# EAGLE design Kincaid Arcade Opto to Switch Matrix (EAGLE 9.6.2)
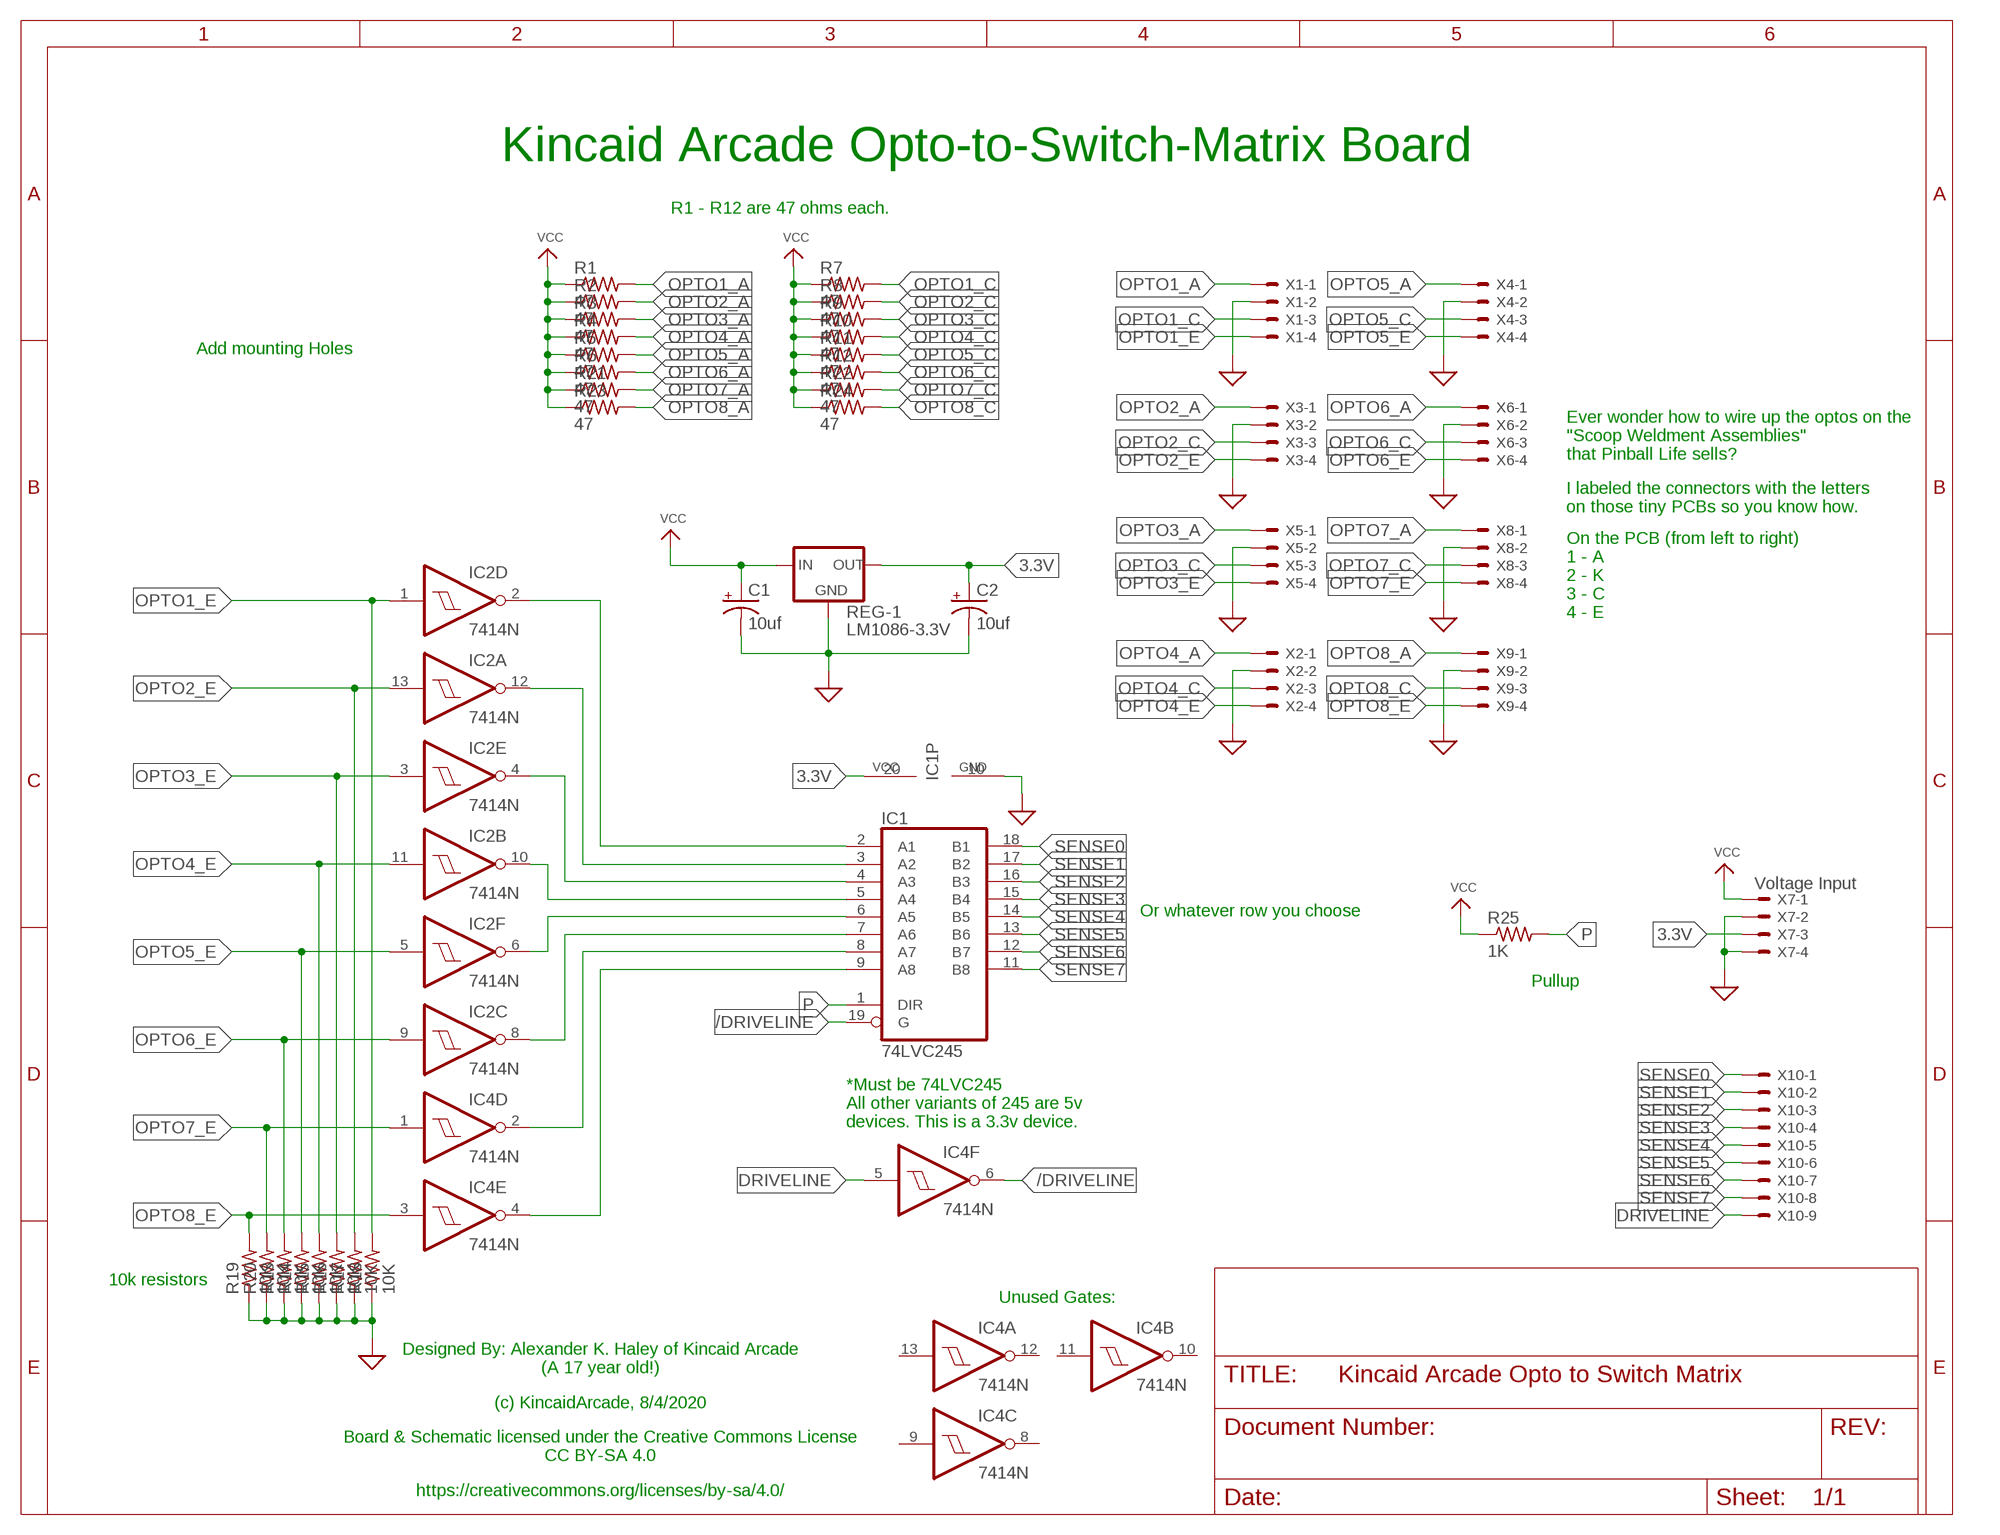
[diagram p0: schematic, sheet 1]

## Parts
C1  10uf  CPOL-USB45181A  [B45181A]
C2  10uf  CPOL-USB45181A  [B45181A]
IC1  74LVC245  74LS245N  [DIL20]
IC2  7414N  [DIL14]
IC4  7414N  [DIL14]
R1  47  R-US_0207/7  [0207/7]
R2  47  R-US_0207/7  [0207/7]
R3  47  R-US_0207/7  [0207/7]
R4  47  R-US_0207/7  [0207/7]
R5  47  R-US_0207/7  [0207/7]
R6  47  R-US_0207/7  [0207/7]
R7  47  R-US_0207/7  [0207/7]
R8  47  R-US_0207/7  [0207/7]
R9  47  R-US_0207/7  [0207/7]
R10  47  R-US_0207/7  [0207/7]
R11  47  R-US_0207/7  [0207/7]
R12  47  R-US_0207/7  [0207/7]
R13  10K  R-US_0207/7  [0207/7]
R14  10K  R-US_0207/7  [0207/7]
R15  10K  R-US_0207/7  [0207/7]
R16  10K  R-US_0207/7  [0207/7]
R17  10K  R-US_0207/7  [0207/7]
R18  10K  R-US_0207/7  [0207/7]
R19  10K  R-US_0207/7  [0207/7]
R20  10K  R-US_0207/7  [0207/7]
R21  47  R-US_0207/7  [0207/7]
R22  47  R-US_0207/7  [0207/7]
R23  47  R-US_0207/7  [0207/7]
R24  47  R-US_0207/7  [0207/7]
R25  1K  R-US_0207/7  [0207/7]
REG-1  LM1086-3.3V  LM1086  [78XXL]
X1  KK-156-4  [KK-156-4]
X2  KK-156-4  [KK-156-4]
X3  KK-156-4  [KK-156-4]
X4  KK-156-4  [KK-156-4]
X5  KK-156-4  [KK-156-4]
X6  KK-156-4  [KK-156-4]
X7  Voltage Input  KK-156-4  [KK-156-4]
X8  KK-156-4  [KK-156-4]
X9  KK-156-4  [KK-156-4]
X10  KK-156-9  [KK-156-9]

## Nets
3.3V: C2.+ IC1.20(VCC) REG-1.OUT X7.3
/DRIVELINE: IC1.19(G) IC4.6(F:O)
DRIVELINE: IC4.5(F:I) X10.9
GND: C1.- C2.- IC1.10(GND) R13.1 R14.1 R15.1 R16.1 R17.1 R18.1 R19.1 R20.1 REG-1.GND X1.2 X2.2 X3.2 X4.2 X5.2 X6.2 X7.2 X7.4 X8.2 X9.2 ; supply symbol labelled SUP
N$1: IC1.9(A8) IC4.4(E:O)
N$2: IC1.8(A7) IC4.2(D:O)
N$3: IC1.7(A6) IC2.8(C:O)
N$4: IC1.6(A5) IC2.6(F:O)
N$5: IC1.5(A4) IC2.10(B:O)
N$6: IC1.4(A3) IC2.4(E:O)
N$7: IC1.3(A2) IC2.12(A:O)
N$8: IC1.2(A1) IC2.2(D:O)
OPTO1_A: R1.2 X1.1
OPTO1_C: R7.2 X1.3
OPTO1_E: IC2.1(D:I) R18.2 X1.4
OPTO2_A: R2.2 X3.1
OPTO2_C: R8.2 X3.3
OPTO2_E: IC2.13(A:I) R17.2 X3.4
OPTO3_A: R3.2 X5.1
OPTO3_C: R9.2 X5.3
OPTO3_E: IC2.3(E:I) R16.2 X5.4
OPTO4_A: R4.2 X2.1
OPTO4_C: R10.2 X2.3
OPTO4_E: IC2.11(B:I) R15.2 X2.4
OPTO5_A: R5.2 X4.1
OPTO5_C: R11.2 X4.3
OPTO5_E: IC2.5(F:I) R14.2 X4.4
OPTO6_A: R6.2 X6.1
OPTO6_C: R12.2 X6.3
OPTO6_E: IC2.9(C:I) R13.2 X6.4
OPTO7_A: R21.2 X8.1
OPTO7_C: R22.2 X8.3
OPTO7_E: IC4.1(D:I) R20.2 X8.4
OPTO8_A: R23.2 X9.1
OPTO8_C: R24.2 X9.3
OPTO8_E: IC4.3(E:I) R19.2 X9.4
P: IC1.1(DIR) R25.2
SENSE0: IC1.18(B1) X10.1
SENSE1: IC1.17(B2) X10.2
SENSE2: IC1.16(B3) X10.3
SENSE3: IC1.15(B4) X10.4
SENSE4: IC1.14(B5) X10.5
SENSE5: IC1.13(B6) X10.6
SENSE6: IC1.12(B7) X10.7
SENSE7: IC1.11(B8) X10.8
VCC: C1.+ R1.1 R2.1 R3.1 R4.1 R5.1 R6.1 R7.1 R8.1 R9.1 R10.1 R11.1 R12.1 R21.1 R22.1 R23.1 R24.1 R25.1 REG-1.IN X7.1
Unconnected: IC4.8(C:O) IC4.9(C:I) IC4.10(B:O) IC4.11(B:I) IC4.12(A:O) IC4.13(A:I)

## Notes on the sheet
- Kincaid Arcade Opto-to-Switch-Matrix Board
- R1 - R12 are 47 ohms each.
- Add mounting Holes
- Ever wonder how to wire up the optos on the
  "Scoop Weldment Assemblies"
  that Pinball Life sells?
- I labeled the connectors with the letters
  on those tiny PCBs so you know how.
- On the PCB (from left to right)
  1 - A
  2 - K
  3 - C
  4 - E
- Or whatever row you choose
- Pullup
- *Must be 74LVC245
  All other variants of 245 are 5v
  devices. This is a 3.3v device.
- 10k resistors
- Unused Gates:
- Designed By: Alexander K. Haley of Kincaid Arcade
  (A 17 year old!)
- (c) KincaidArcade, 8/4/2020
- Board & Schematic licensed under the Creative Commons License
  CC BY-SA 4.0
- https://creativecommons.org/licenses/by-sa/4.0/

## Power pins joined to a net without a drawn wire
GND: IC2.7(P:GND) IC4.7(P:GND)
VCC: IC2.14(P:VCC) IC4.14(P:VCC)

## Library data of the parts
C1 C2 = rcl:CPOL-US: POLARIZED CAPACITOR, American symbol; SPICEPREFIX: C
IC1 = 74xx-us:74*245: Octal BUS TRANSCEIVER, 3-state
IC2 IC4 = 74xx-us:74*14: Hex schmitt trigger INVERTER
R1-R24 = resistor:R-US_: RESISTOR, American symbol
R25 = rcl:R-US_: RESISTOR, American symbol; SPICEPREFIX: R
REG-1 = OLD AND OBSOLETE ARCADE PARTS:LM1086
X1-X9 = con-molex:KK-156-4: KK 156 HEADER Source: http://www.molex.com/pdm_docs/sd/026604100_sd.pdf; MF: MOLEX; OC_FARNELL: unknown; OC_NEWARK: unknown
X10 = con-molex:KK-156-9: KK 156 HEADER Source: http://www.molex.com/pdm_docs/sd/026604100_sd.pdf; MF: MOLEX; OC_FARNELL: unknown; OC_NEWARK: unknown

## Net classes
0 default: width 0.406 mm, clearance 0.406 mm

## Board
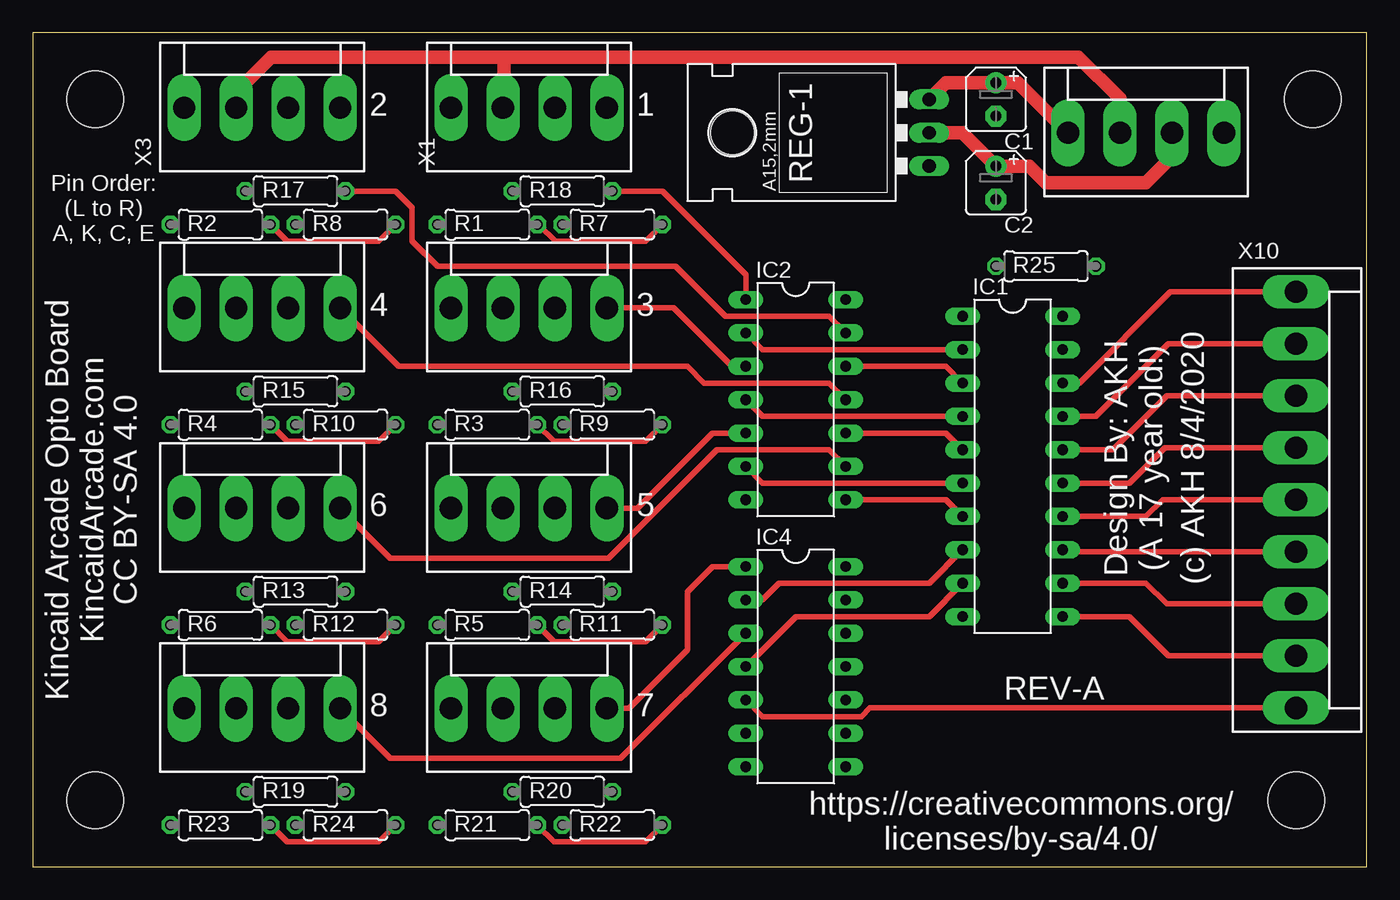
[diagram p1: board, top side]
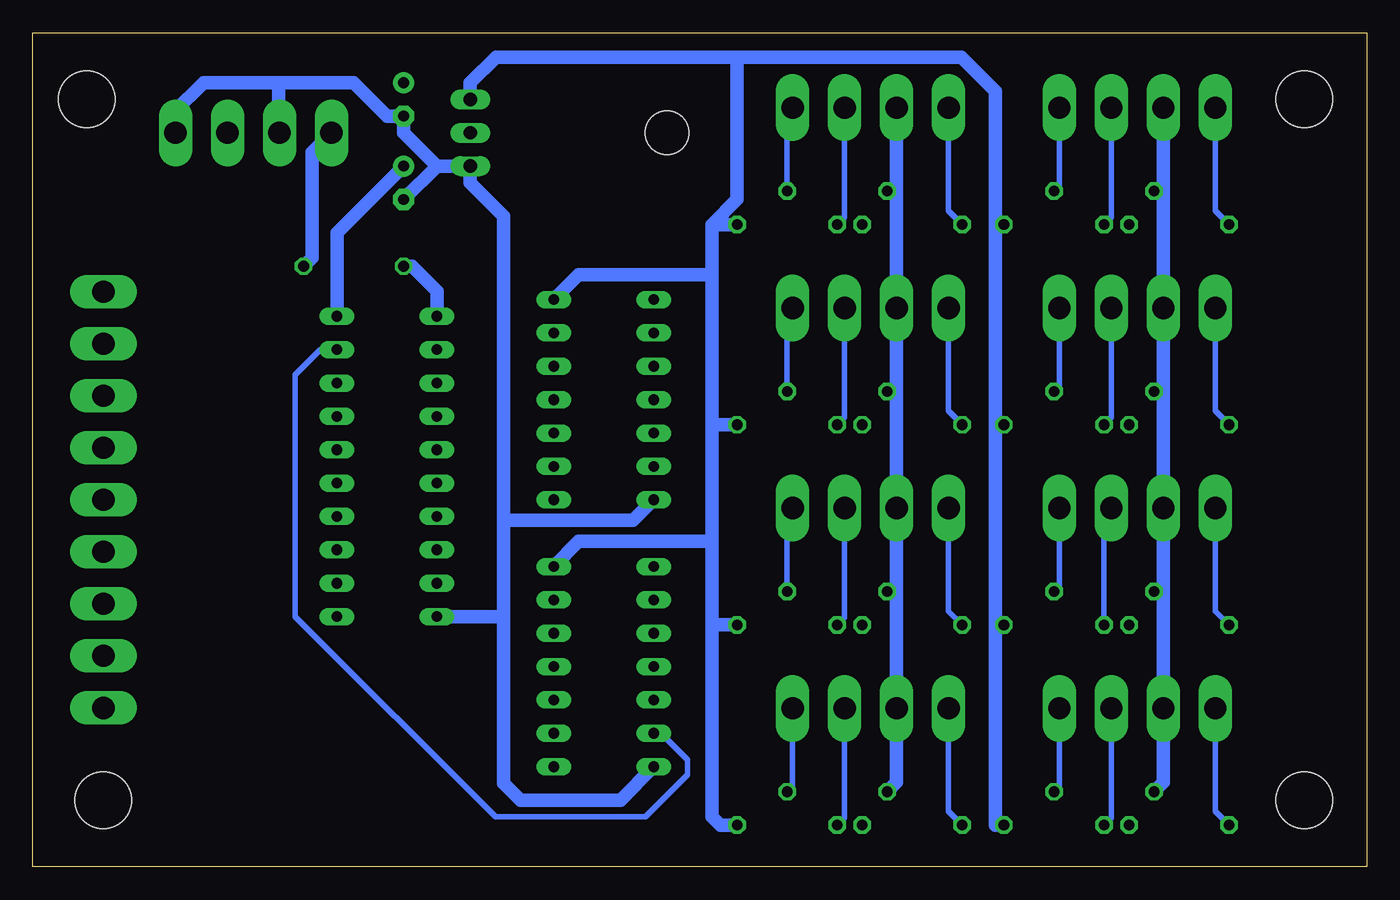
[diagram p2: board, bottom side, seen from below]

Size 101.58 x 63.49 mm. Coordinates in mm from the lower left corner, seen from the top.
Outline: 0,0 101.58,0 101.58,63.49 0,63.49 0,0
Copper layers (1*16): Top 0.035mm / dielectric 1.5mm / Bottom 0.035mm
Design rules "default": minimum track width 6mil, minimum drill 0.35mm, track to track 6mil, track to pad 6mil, pad to pad 6mil, via to via 6mil, smd to smd 6mil, copper to edge 40mil, drill to drill 6mil, minimum pad ring 10mil, minimum via ring 8mil, stop-mask expansion 4mil, vias tented up to drill 0mil, thermal gap 10mil
Holes 4.32 mm at 4.76,58.42 4.76,5.08 97.47,58.42 96.2,5.08

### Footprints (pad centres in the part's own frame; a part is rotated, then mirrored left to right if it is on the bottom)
B45181A = drill 0.813 pad 1.6: + -1.27,0 | drill 0.813 pad 1.6 octagon: - 1.27,0
DIL20 = drill 0.813 long: 1 -11.43,-3.81; 2 -8.89,-3.81; 3 -6.35,-3.81; 4 -3.81,-3.81; 5 -1.27,-3.81; 6 1.27,-3.81; 7 3.81,-3.81; 8 6.35,-3.81; 9 8.89,-3.81; 10 11.43,-3.81; 11 11.43,3.81; 12 8.89,3.81; 13 6.35,3.81; 14 3.81,3.81; 15 1.27,3.81; 16 -1.27,3.81; 17 -3.81,3.81; 18 -6.35,3.81; 19 -8.89,3.81; 20 -11.43,3.81
DIL14 = drill 0.813 long: 1 -7.62,-3.81; 2 -5.08,-3.81; 3 -2.54,-3.81; 4 0,-3.81; 5 2.54,-3.81; 6 5.08,-3.81; 7 7.62,-3.81; 8 7.62,3.81; 9 5.08,3.81; 10 2.54,3.81; 11 0,3.81; 12 -2.54,3.81; 13 -5.08,3.81; 14 -7.62,3.81
0207/7 = drill 0.813 octagon: 1 -3.81,0; 2 3.81,0
78XXL = drill 1.016 long: GND -2.54,-3.81; IN 2.54,-3.81; OUT 0,-3.81 | hole 3.302: 0,11.176
KK-156-4 = drill 1.7 pad 2.184 long: 1 -5.94,0; 2 -1.98,0; 3 1.98,0; 4 5.94,0
KK-156-9 = drill 1.7 pad 2.184 long: 1 -15.84,0; 2 -11.88,0; 3 -7.92,0; 4 -3.96,0; 5 0,0; 6 3.96,0; 7 7.92,0; 8 11.88,0; 9 15.84,0

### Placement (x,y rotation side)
C1  73.34,58.42 270 top
C2  73.34,52.07 270 top
IC1  74.61,30.48 270 top
IC2  58.1,35.56 270 top
IC4  58.1,15.24 270 top
R1  34.61,48.9 180 top
R2  14.29,48.9 180 top
R3  34.61,33.66 180 top
R4  14.29,33.66 180 top
R5  34.61,18.41 180 top
R6  14.29,18.41 180 top
R7  44.13,48.9 180 top
R8  23.81,48.9 180 top
R9  44.13,33.66 180 top
R10  23.81,33.66 180 top
R11  44.13,18.41 180 top
R12  23.81,18.41 180 top
R13  20,20.95 0 top
R14  40.32,20.95 0 top
R15  20,36.2 0 top
R16  40.32,36.2 0 top
R17  20,51.44 0 top
R18  40.32,51.44 0 top
R19  20,5.71 0 top
R20  40.32,5.71 0 top
R21  34.61,3.17 180 top
R22  44.13,3.17 180 top
R23  14.29,3.17 180 top
R24  23.81,3.17 180 top
R25  77.15,45.72 180 top
REG-1  64.45,55.88 90 top
X1  37.78,57.78 0 top
X2  17.46,42.55 0 top
X3  17.46,57.78 0 top
X4  37.78,27.3 0 top
X5  37.78,42.55 0 top
X6  17.46,27.3 0 top
X7  84.77,55.88 0 top
X8  37.78,12.06 0 top
X9  17.46,12.06 0 top
X10  96.2,27.94 270 top

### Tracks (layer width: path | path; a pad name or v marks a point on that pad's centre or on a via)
3.3V
  Top 1.016: REG-1.OUT 70.8,55.88 C2.+ 75.88,53.34 77.15,52.07 84.77,52.07 86.75,54.05 X7.3
  Bottom 1.016: C2.+ 78.42,48.26 IC1.20
/DRIVELINE
  Bottom 0.406: IC4.6 53.74,10.16 51.73,8.15 51.73,7.01 54.93,3.81 66.36,3.81 81.6,19.05 81.6,37.47 79.69,39.37 IC1.19
DRIVELINE
  Top 0.406: X10.9 63.77,12.1 63.1,11.43 55.56,11.43 IC4.5
GND
  Top 1.016: X7.2 82.79,58.49 79.64,61.65 35.88,61.65 | 35.88,61.65 18.15,61.65 15.48,58.98 X3.2 | 35.88,61.65 35.88,57.86 X1.2
  Bottom 1.016: 70.8,53.34 REG-1.GND 68.26,52.07 65.72,49.53 65.72,26.36 | 70.8,53.34 C2.- | 70.8,53.34 73.34,55.88 C1.- 74.61,57.15 77.15,59.69 82.87,59.69 | X7.4 90.85,56.01 90.85,57.43 88.58,59.69 82.87,59.69 | 82.87,59.69 82.87,55.95 X7.2 | 65.72,26.36 65.72,19.05 | 65.72,19.05 65.72,6.35 64.45,5.08 56.83,5.08 IC4.7 | 65.72,26.36 55.87,26.36 IC2.7 | IC1.10 65.72,19.05 | X3.2 15.48,51.44 | 15.48,51.44 X2.2 15.48,36.2 | R17.1 15.48,51.44 | X1.2 35.8,51.44 | 35.8,51.44 X5.2 35.8,36.2 | R18.1 35.8,51.44 | 35.8,36.2 X4.2 35.8,20.95 | R16.1 35.8,36.2 | 15.48,36.2 X6.2 15.48,20.95 | R15.1 15.48,36.2 | 15.48,20.95 X9.2 15.48,6.42 R19.1 | R13.1 15.48,20.95 | 35.8,20.95 X8.2 35.8,6.42 R20.1 | R14.1 35.8,20.95
N$1
  Top 0.406: IC4.4 58.1,19.05 68.26,19.05 IC1.9
N$2
  Top 0.406: IC4.2 55.56,20.32 56.83,21.59 68.26,21.59 IC1.8
N$3
  Top 0.406: IC2.8 69.53,27.94 IC1.7
N$4
  Top 0.406: IC2.6 55.56,29.21 IC1.6
N$5
  Top 0.406: IC2.10 69.53,33.02 IC1.5
N$6
  Top 0.406: IC2.4 55.56,34.29 IC1.4
N$7
  Top 0.406: IC2.12 69.53,38.1 IC1.3
N$8
  Top 0.406: IC2.2 55.56,39.37 IC1.2
OPTO1_A
  Bottom 0.406: X1.1 31.84,49.94 R1.2
OPTO1_C
  Bottom 0.406: X1.3 39.76,49.45 R7.2
OPTO1_E
  Top 0.406: IC2.1 54.29,45.09 47.94,51.44 R18.2
  Bottom 0.406: X1.4 44.13,57.38 R18.2
OPTO2_A
  Bottom 0.406: X3.1 11.52,49.94 R2.2
OPTO2_C
  Bottom 0.406: X3.3 19.44,49.45 R8.2
OPTO2_E
  Top 0.406: IC2.13 60.64,41.91 52.74,41.91 48.95,45.7 30.81,45.7 28.89,47.62 28.89,50.16 27.62,51.44 R17.2
  Bottom 0.406: X3.4 23.4,51.84 R17.2
OPTO3_A
  Bottom 0.406: X5.1 31.84,34.7 R3.2
OPTO3_C
  Bottom 0.406: X5.3 39.76,34.22 R9.2
OPTO3_E
  Top 0.406: X5.4 48.8,42.55 53.25,38.1 IC2.3
  Bottom 0.406: X5.4 44.13,42.13 R16.2
OPTO4_A
  Bottom 0.406: X2.1 11.52,34.7 R4.2
OPTO4_C
  Bottom 0.406: X2.3 19.44,34.22 R10.2
OPTO4_E
  Top 0.406: X2.4 27.85,38.1 49.85,38.1 51.12,36.83 60.64,36.83 IC2.11
  Bottom 0.406: X2.4 23.4,36.6 R15.2
OPTO5_A
  Bottom 0.406: X4.1 31.84,19.46 R5.2
OPTO5_C
  Bottom 0.406: X4.3 39.76,18.98 R11.2
OPTO5_E
  Top 0.406: X4.4 46.04,27.3 51.75,33.02 IC2.5
  Bottom 0.406: X4.4 44.13,26.89 R14.2
OPTO6_A
  Bottom 0.406: X6.1 11.52,19.46 R6.2
OPTO6_C
  Bottom 0.406: X6.3 20,26.75 R12.2
OPTO6_E
  Top 0.406: X6.4 27.21,23.5 43.85,23.5 52.11,31.75 60.64,31.75 IC2.9
  Bottom 0.406: X6.4 23.4,21.36 R13.2
OPTO7_A
  Bottom 0.406: X8.1 31.84,4.22 R21.2
OPTO7_C
  Bottom 0.406: X8.3 39.76,3.73 R22.2
OPTO7_E
  Top 0.406: IC4.1 51.75,22.86 49.85,20.95 49.85,16.51 45.4,12.06 X8.4
  Bottom 0.406: X8.4 43.72,6.12 R20.2
OPTO8_A
  Bottom 0.406: X9.1 11.52,4.22 R23.2
OPTO8_C
  Bottom 0.406: X9.3 19.44,3.73 R24.2
OPTO8_E
  Top 0.406: X9.4 27.21,8.26 44.77,8.26 IC4.3
  Bottom 0.406: X9.4 23.4,6.12 R19.2
P
  Bottom 1.016: R25.2 72.71,45.72 70.8,43.81 IC1.1
SENSE0
  Top 0.406: IC1.18 79.69,36.83 86.64,43.78 X10.1
SENSE1
  Top 0.406: X10.2 86.49,39.82 80.96,34.29 IC1.17
SENSE2
  Top 0.406: IC1.16 82.23,31.75 86.34,35.86 X10.3
SENSE3
  Top 0.406: X10.4 86.19,31.9 83.5,29.21 IC1.15
SENSE4
  Top 0.406: IC1.14 84.77,26.67 86.04,27.94 X10.5
SENSE5
  Top 0.406: X10.6 78.57,23.98 IC1.13
SENSE6
  Top 0.406: X10.7 86.34,20.02 84.77,21.59 IC1.12
SENSE7
  Top 0.406: X10.8 86.49,16.06 83.5,19.05 IC1.11
VCC
  Top 0.406: R1.1 38.53,48.9 39.8,47.62 46.67,47.62 R7.1 | R5.1 39.69,17.14 46.67,17.14 R11.1 | R2.1 19.37,47.62 26.35,47.62 R8.1 | R6.1 19.37,17.14 26.35,17.14 R12.1 | R3.1 39.69,32.38 46.67,32.38 R9.1 | R21.1 39.69,1.91 46.67,1.91 R22.1 | R4.1 19.37,32.38 26.35,32.38 R10.1 | R23.1 19.37,1.91 26.35,1.91 R24.1
  Top 1.016: REG-1.IN 69.53,59.69 C1.+ 75.02,59.69 X7.1
  Bottom 1.016: REG-1.IN 68.26,59.69 66.31,61.65 47.94,61.65 | 28.26,18.41 28.26,3.17 R24.1 | 28.26,18.41 28.26,33.66 | 28.26,33.66 28.26,48.9 | 28.26,48.9 28.26,59.05 30.85,61.65 47.94,61.65 | 49.85,48.9 49.85,45.09 | 49.85,45.09 49.85,33.66 | 49.85,33.66 49.85,24.77 | 49.85,24.77 49.85,18.41 | 49.85,18.41 49.85,3.81 49.21,3.17 R22.1 | 49.85,45.09 60.01,45.09 IC2.14 | 49.85,24.77 60.01,24.77 IC4.14 | R11.1 49.85,18.41 | R12.1 28.26,18.41 | R10.1 28.26,33.66 | R9.1 49.85,33.66 | R7.1 49.85,48.9 | R8.1 28.26,48.9 | X7.1 80.33,54.38 80.33,46.35 R25.1 | 49.85,48.9 47.94,50.8 47.94,61.65

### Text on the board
tPlace: 2 | 1 | Pin Order: | (L to R) | A, K, C, E | 4 | 3 | Design By: AKH / (A 17 year old!) | (c) AKH 8/4/2020 | Kincaid Arcade Opto Board | KincaidArcade.com | CC BY-SA 4.0 | 6 | 5 | REV-A | 8 | 7 | https://creativecommons.org/ / licenses/by-sa/4.0/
